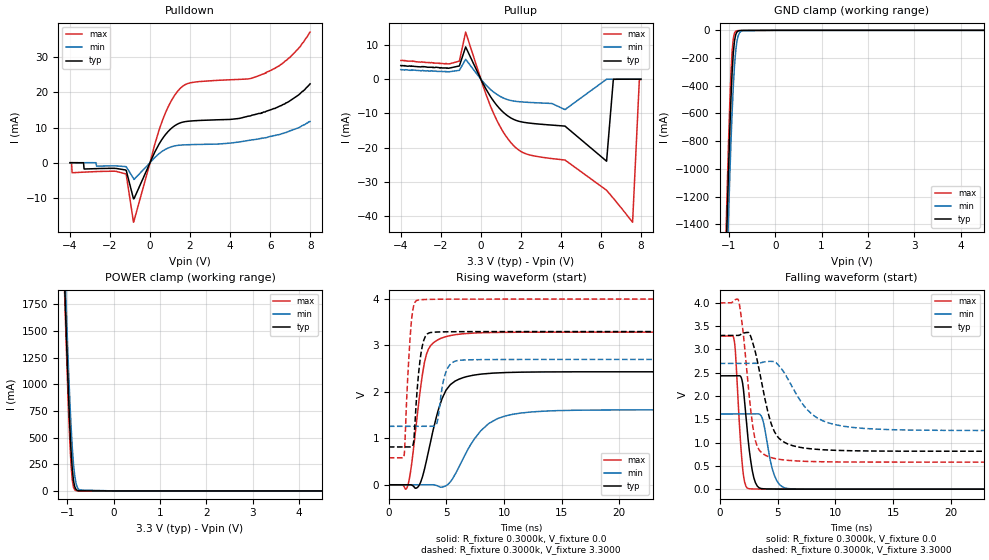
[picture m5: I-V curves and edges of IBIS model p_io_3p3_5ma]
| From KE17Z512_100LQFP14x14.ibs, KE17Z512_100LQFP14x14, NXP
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[Model] p_io_3p3_5ma
|   Model p_io_3p3_5ma
| This model was characterised for following simulation conditions:
| External (pad) voltage:
|   - Typ: 3.3V,   - Min: 2.7V,   - Max: 4.0V
| Library cells for typ/min/max conditions are connected as defined below:
|  pad - External Pad
|  ipp_do_lv - Core Input
|  ipp_obe_lv - Output Buffer Enable
|  abt_close_nor_rst_mv - vdde
|  dvdd - dvdd
|  dvss - dvss
|  esd_boost - vdde
|  ipp_ina_280_mv - NC
|  ipp_ina_40_a_mv - NC
|  ipp_ina_40_b_mv - NC
|  ipp_ina_40_c_mv - NC
|  ipp_ina_40_d_mv - NC
|  ipp_ina_40_e_mv - NC
|  ipp_ina_40_f_mv - NC
|  ipp_ina_40_g_mv - NC
|  ipp_ina_40_h_mv - NC
|  ipp_ind_lv - NC
|  vdde - vdde
|  vsse - vsse
| All other pins connected to ground
Model_type I/O
Polarity   Non-Inverting
Enable   Active-High
Vinl =   0.9900V
Vinh =   2.3100V
Vmeas =  1.6500V
Cref =   50.0000F
C_comp   1.4830pF   1.4157pF   1.5731pF
[Model Spec]
| variable   typ   min   max
Vinh   2.3100V   1.8900V   2.8000V
Vinl   0.9900V   0.8100V   1.2000V
S_overshoot_high   3.6000V   3.0000V   4.3000V
S_overshoot_low   -0.3000V   -0.3000V   -0.3000V
Vmeas   1.6500V   1.3500V   2.0000V
[Temperature Range]   25.0000   0.1250k   -40.0000
[Voltage Range]   3.3000V   2.7000V   4.0000V
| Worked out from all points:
|   slope of the pulldown table from 0 to 0.495 V, typ, clamps not added: 86.7 ohm
|   slope of the pullup table from 0 to 0.495 V, typ, clamps not added: 95.4 ohm
|   GND clamp passes 1 mA (typ) near -0.73 V on its own axis
|   rising waveform, R_fixture 0.3000k, V_fixture 0.0: 20-80 % time 1.56ns typ, 2.59ns min, 1ns max; typ from 0 V to 2.43 V
|   rising waveform, R_fixture 0.3000k, V_fixture 3.3000: 20-80 % time 511ps typ, 598ps min, 437ps max; typ from 0.814 V to 3.3 V
|   falling waveform, R_fixture 0.3000k, V_fixture 0.0: 20-80 % time 630ps typ, 792ps min, 473ps max; typ from 2.43 V to 0 V
|   falling waveform, R_fixture 0.3000k, V_fixture 3.3000: 20-80 % time 1.38ns typ, 2.53ns min, 865ps max; typ from 3.3 V to 0.814 V
[Pulldown]
|Voltage   I(typ)   I(min)   I(max)
-4V       10uA       10uA       -80uA
-3.922V   10uA       10uA       -90uA
-3.896V   10uA       10uA       -2.85mA
-3.324V   -20uA      10uA       -2.68mA
-3.298V   -1.79mA    0A         -2.68mA
-1.218V   -2.07mA    -1.098mA   -3.166mA
-828mV    -10.24mA   -4.449mA   -16.89mA
576mV     6.453mA    3.116mA    11.33mA
1.46V     11.2mA     4.969mA    20.82mA
5.802V    14.6mA     7.1mA      25.5mA
6.972V    17.5mA     9mA        29.8mA
8V        22.4mA     11.7mA     37.1mA
[Pullup]
|Voltage   I(typ)   I(min)   I(max)
-4V       4mA        2.8mA      5.5mA
-1.074V   3.89mA     2.61mA     5.3mA
-762mV    9.447mA    5.831mA    13.78mA
460mV     -4.878mA   -2.876mA   -7.555mA
1.552V    -11.47mA   -6.274mA   -18.86mA
2.384V    -12.78mA   -6.754mA   -22.03mA
4.204V    -13.69mA   -8.866mA   -23.6mA
6.284V    -23.94mA   10uA       -32.43mA
6.622V    -20uA      10uA       -34.78mA
7.584V    20uA       10uA       -41.76mA
7.922V    10uA       10uA       -90uA
8V        20uA       10uA       -80uA
[GND_clamp]
|Voltage   I(typ)   I(min)   I(max)
-4V       -46.16A    -46.12A    -46.24A
-1.062V   -1.635A    -1.959A    -1.443A
-1.036V   -1.319A    -1.649A    -1.12A
-1.01V    -1.02A     -1.353A    -816.5mA
-958mV    -503mA     -819.8mA   -315.6mA
-932mV    -305.3mA   -593.7mA   -150.8mA
-906mV    -162.1mA   -403mA     -57.82mA
-880mV    -74.91mA   -253.4mA   -19.32mA
-828mV    -12.56mA   -79.29mA   -3.027mA
-776mV    -2.422mA   -20.15mA   -1.541mA
-698mV    -671uA     -2.492mA   -991.9uA
8V        0A         0A         0A
[POWER_clamp]
|Voltage   I(typ)   I(min)   I(max)
-4V       49.34A     49.12A     49.54A
-1.074V   2.177A     2.376A     2.076A
-1.048V   1.824A     2.037A     1.712A
-1.022V   1.484A     1.709A     1.36A
-970mV    862.3mA    1.105A     718.6mA
-918mV    371.6mA    601.7mA    237.9mA
-892mV    203.6mA    404mA      100.5mA
-866mV    96.41mA    250.6mA    34.26mA
-814mV    15.77mA    76.07mA    3.222mA
-736mV    1.005mA    9.029mA    404.2uA
0V        65.13pA    866.3pA    64.14pA
8V        0A         0A         0A
[Ramp]
| variable   typ   min   max
dV/dt_r  1.4599/1.5561n   0.9681/2.5857n   1.9724/1.0024n
dV/dt_f  1.4917/1.3843n   0.8648/2.5327n   2.0518/0.8652n
R_load = 0.3000k
[Rising Waveform]
R_fixture= 0.3000k
V_fixture= 0.0
V_fixture_min= 0.0
V_fixture_max= 0.0
|time   V(typ)   V(min)   V(max)
0s        63.99pV    15.7nV     179.8pV
1.615ns   -24.02uV   -4.806uV   -37.98mV
1.929ns   -1.233mV   2.665uV    356mV
2.573ns   -32.41mV   297.8nV    1.736V
3.263ns   520.1mV    -47.39uV   2.813V
4.283ns   1.606V     -31.25mV   3.126V
4.851ns   1.979V     -33.4mV    3.184V
7.975ns   2.382V     1.163V     3.274V
10.79ns   2.422V     1.52V      3.285V
40ns      2.433V     1.613V     3.287V
[Rising Waveform]
R_fixture= 0.3000k
V_fixture= 3.3000
V_fixture_min= 2.7000
V_fixture_max= 4.0000
|time   V(typ)   V(min)   V(max)
0s        813.9mV    1.259V     580.3mV
1.312ns   813.9mV    1.259V     615.9mV
1.909ns   813.5mV    1.259V     3.396V
2.155ns   935.2mV    1.259V     3.859V
2.447ns   2.02V      1.259V     3.973V
3.167ns   3.197V     1.259V     3.991V
4.103ns   3.289V     1.291V     3.996V
4.902ns   3.295V     2.395V     3.998V
5.928ns   3.297V     2.674V     3.999V
40ns      3.3V       2.7V       4V
[Falling Waveform]
R_fixture= 0.3000k
V_fixture= 0.0
V_fixture_min= 0.0
V_fixture_max= 0.0
|time   V(typ)   V(min)   V(max)
0s        2.433V     1.613V     3.287V
1.234ns   2.433V     1.613V     3.226V
1.965ns   2.3V       1.613V     492.7mV
2.461ns   1.058V     1.613V     14.22mV
2.828ns   387.7mV    1.613V     4.807mV
3.258ns   62.91mV    1.617V     2.833mV
3.73ns    8.162mV    1.486V     1.781mV
4.733ns   2.326mV    294.1mV    860uV
5.933ns   1.016mV    12.04mV    425.3uV
40ns      199.7nV    534nV      86.5nV
[Falling Waveform]
R_fixture= 0.3000k
V_fixture= 3.3000
V_fixture_min= 2.7000
V_fixture_max= 4.0000
|time   V(typ)   V(min)   V(max)
0s        3.3V       2.7V       4V
1.638ns   3.301V     2.7V       4.045V
2.025ns   3.348V     2.7V       3.377V
2.531ns   3.359V     2.7V       2.062V
2.991ns   3.028V     2.7V       1.153V
4.376ns   1.469V     2.745V     683.5mV
5.359ns   1.042V     2.578V     633.7mV
7.99ns    863.2mV    1.605V     592.7mV
10.75ns   827.9mV    1.349V     583.6mV
40ns      813.9mV    1.259V     580.3mV
